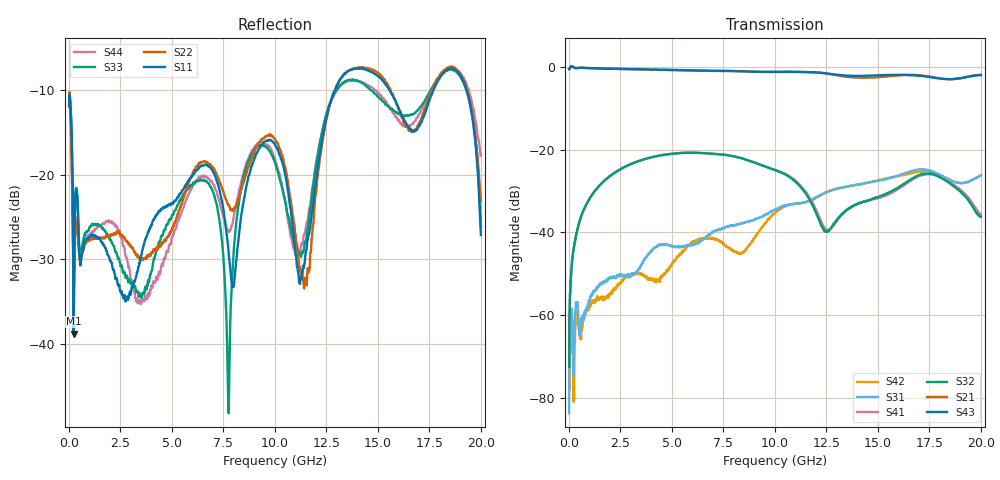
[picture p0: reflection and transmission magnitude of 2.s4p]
!Keysight Technologies,N5225A,MY51451420,A.10.40.12
!Date: Tuesday, October 13, 2015 10:33:35
!Correction: S11(Full 4 Port(1,2,3,4))
!S12(Full 4 Port(1,2,3,4))
!S13(Full 4 Port(1,2,3,4))
!S14(Full 4 Port(1,2,3,4))
!S21(Full 4 Port(1,2,3,4))
!S22(Full 4 Port(1,2,3,4))
!S23(Full 4 Port(1,2,3,4))
!S24(Full 4 Port(1,2,3,4))
!S31(Full 4 Port(1,2,3,4))
!S32(Full 4 Port(1,2,3,4))
!S33(Full 4 Port(1,2,3,4))
!S34(Full 4 Port(1,2,3,4))
!S41(Full 4 Port(1,2,3,4))
!S42(Full 4 Port(1,2,3,4))
!S43(Full 4 Port(1,2,3,4))
!S44(Full 4 Port(1,2,3,4))
!S4P File: Measurements: <S11,S12,S13,S14>,
!<S21,S22,S23,S24>,
!<S31,S32,S33,S34>,
!<S41,S42,S43,S44>:
# Hz S  dB  R 50
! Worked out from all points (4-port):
!   1999 points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, 20 MHz to 20 GHz, reference 50 ohm
!   strongest paths, dB at 20 MHz, 5.01 GHz, 10.01 GHz, 15.01 GHz, 20 GHz:
!     S43: -0.5, -0.8, -1.2, -2.1, -2.0
!     S21: -0.5, -0.8, -1.3, -2.5, -2.0
!     S32: -72.5, -21.0, -24.9, -31.4, -36.2
!     S41: -68.4, -21.0, -24.9, -31.7, -35.7
!     S31: -83.7, -43.4, -34.5, -27.6, -26.2
!     S42: -65.7, -47.6, -35.3, -27.4, -26.1
!   lowest |S11| = -38.7 dB at 240 MHz (marker M1), VSWR 1.02, Z = 50.3 - j1.12 ohm
!   |S11| at or under -10 dB: start of sweep to 12.92 GHz; 15.57 GHz to 17.7 GHz (2.132 GHz wide, 12.8 % of centre); 19.3 GHz to end of sweep
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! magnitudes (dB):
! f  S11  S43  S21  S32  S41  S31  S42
! 20 MHz  -11.8  -0.5  -0.5  -72.5  -68.4  -83.7  -65.7
! 240 MHz  -38.7  -0.1  -0.1  -44.1  -44.0  -74.7  -78.7
! 5.24 GHz  -22.8  -0.8  -0.8  -20.9  -20.9  -43.6  -46.2
! 7.75 GHz  -28.8  -1.0  -1.0  -21.4  -21.4  -38.6  -43.7
! 11.48 GHz  -29.5  -1.2  -1.3  -30.4  -30.1  -32.7  -32.7
! 13.42 GHz  -8.0  -2.1  -2.4  -34.9  -34.9  -29.0  -29.0
! 20 GHz  -27.1  -2.0  -2.0  -36.2  -35.7  -26.2  -26.1
